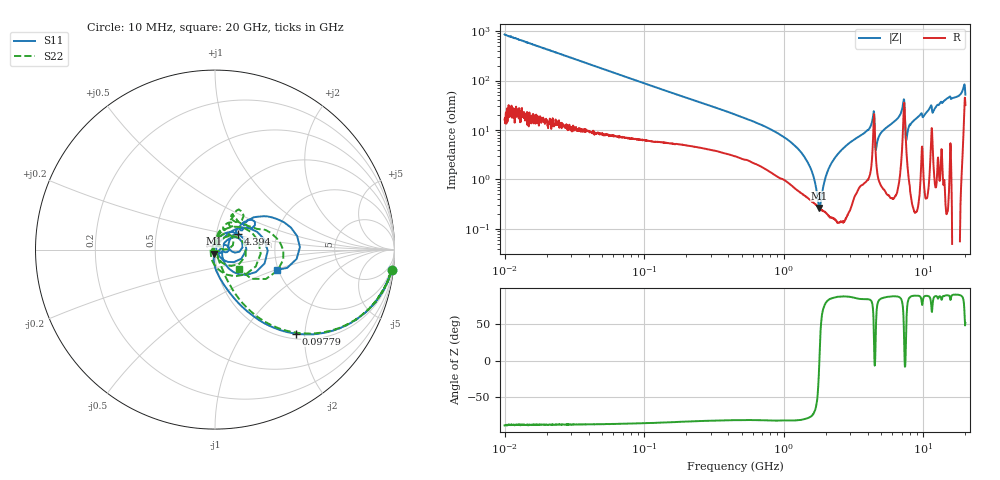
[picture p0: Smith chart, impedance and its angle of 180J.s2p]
!Keysight Technologies,P5008B,MY61100088,A.16.20.02
!Date: Monday, November 06, 2023 16:32:38
!Correction: S11(C  2-Port  )
!S21(C  2-Port  )
!S12(C  2-Port  )
!S22(C  2-Port  )
!S2P File: Measurements: S11, S21, S12, S22:Log Frequency Sweep
# Hz S  dB  R 50
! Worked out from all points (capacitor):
!   1601 points, 10 MHz to 20 GHz, reference 50 ohm
!   read as one part in series: C = 18.7 pF near 10.39 MHz
!   lowest |Z| = 265 mohm at 1.799 GHz (marker M1)
!   series resonance near 1.797 GHz, so ESL is about 420 pH
!   S11 on the Smith chart (normalised r, x): 10 MHz: 1, -17; 97.79 MHz: 1.11, -1.80; 4.394 GHz: 1.27, +0.23; 20 GHz: 1.97, -0.52
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1e7  -0.08 -6.7  -18.69 82.2  -18.69 82.3  -0.08 -6.7
3.555162e7  -0.79 -22.0  -8.55 65.6  -8.56 65.6  -0.81 -22.0
9.779328e7  -3.73 -46.0  -2.87 40.0  -2.88 40.0  -3.84 -45.9
1.263918e8  -5.06 -52.2  -2.06 33.3  -2.06 33.3  -5.23 -51.9
4.472136e8  -13.46 -74.7  -0.44 11.0  -0.44 11.0  -14.48 -67.9
1.589917e9  -29.10 -100.8  -0.07 -0.1  -0.07 -0.1  -31.78 -77.1
1.798938e9  -32.58 -102.4  -0.06 -1.1  -0.06 -1.1  -35.78 -85.4
2.461408e9  -46.47 -172.1  -0.07 -3.9  -0.07 -3.9  -44.28 -174.2
3.242246e9  -29.07 101.4  -0.16 -6.4  -0.16 -6.4  -40.87 124.7
4.394274e9  -16.09 34.8  -1.10 -13.7  -1.11 -13.8  -16.34 23.6
4.878388e9  -41.79 21.1  -0.06 -9.0  -0.06 -9.1  -38.19 5.2
5.652411e9  -30.87 66.4  -0.03 -12.2  -0.04 -12.3  -29.33 66.9
7.202016e9  -11.88 22.9  -1.68 -24.1  -1.68 -24.1  -12.90 24.8
7.957563e9  -27.36 -19.5  -0.06 -14.9  -0.06 -14.9  -32.20 -179.8
8.424378e9  -32.46 -13.1  -0.01 -17.3  -0.01 -17.3  -36.49 163.5
9.39702e9  -27.62 23.5  -0.02 -21.4  -0.02 -21.4  -30.80 96.3
1.013912e10  -27.44 3.1  -0.03 -22.4  -0.03 -22.4  -32.89 116.7
1.104427e10  -20.93 38.0  -0.10 -27.1  -0.10 -27.0  -21.79 69.0
1.197321e10  -21.17 27.5  -0.09 -26.6  -0.10 -26.6  -22.74 81.3
1.475668e10  -12.29 42.0  -0.22 -36.8  -0.22 -36.8  -12.35 61.4
1.862442e10  -11.68 40.6  -0.47 -53.3  -0.47 -53.3  -12.36 32.0
2e10  -8.78 -18.2  -2.86 -42.5  -2.86 -42.5  -15.12 -39.0
